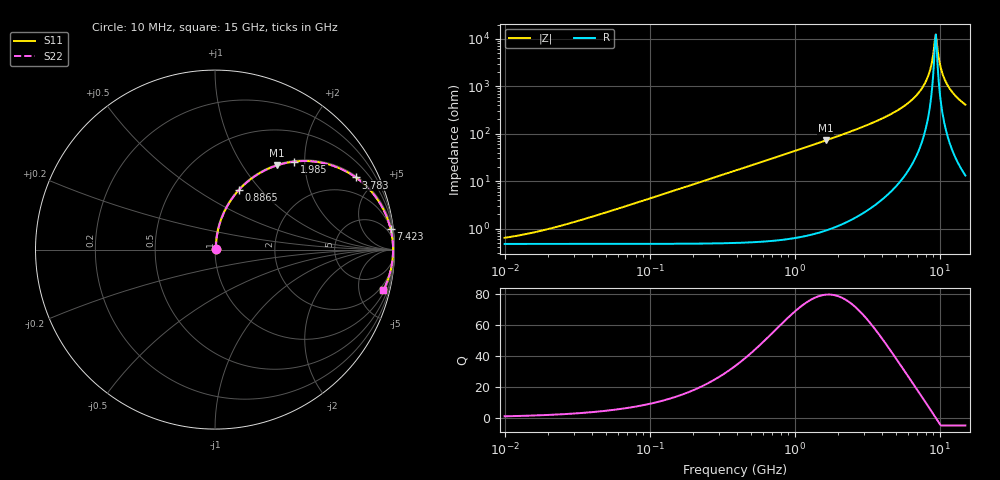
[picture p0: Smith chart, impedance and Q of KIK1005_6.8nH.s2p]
!version-3
!date-01.2023
!Series
# Hz S RI R 50
!Freq ReS11 ImS11 ReS21 ImS21 ReS12 ImS12 ReS22 ImS22
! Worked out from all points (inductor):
!   500 points, 10 MHz to 15 GHz, reference 50 ohm
!   read as one part in series: L = 6.8 nH near 33.75 MHz
!   highest Q = 79.5 at 1.641 GHz (marker M1), where L = 7.01 nH
!   self-resonance near 9.248 GHz
!   S11 on the Smith chart (normalised r, x): 10 MHz: 1.01, +0.01; 886.5 MHz: 1.01, +0.76; 1.985 GHz: 1.02, +1.78; 3.783 GHz: 1.07, +3.86; 7.423 GHz: 2, +17; 15 GHz: 1.26, -8.18
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1e7  0.00474 0.00423  0.9953 -0.00423  0.9953 -0.00423  0.00474 0.00423
3.424937e7  0.00493 0.0145  0.9951 -0.0145  0.9951 -0.0145  0.00493 0.0145
1.155953e8  0.00714 0.0488  0.9929 -0.0488  0.9929 -0.0488  0.00714 0.0488
3.901468e8  0.0317 0.1609  0.9683 -0.1609  0.9683 -0.1609  0.0317 0.1609
8.864682e8  0.1313 0.33  0.8687 -0.33  0.8687 -0.33  0.1313 0.33
1.316788e9  0.2506 0.4269  0.7494 -0.4269  0.7494 -0.4269  0.2506 0.4269
1.64055e9  0.3452 0.4692  0.6548 -0.4692  0.6548 -0.4692  0.3452 0.4692
1.984876e9  0.4416 0.4903  0.5584 -0.4903  0.5584 -0.4903  0.4416 0.4903
3.782592e9  0.7842 0.4022  0.2158 -0.4022  0.2158 -0.4022  0.7842 0.4022
4.444302e9  0.8517 0.3444  0.1483 -0.3444  0.1483 -0.3444  0.8517 0.3444
6.04598e9  0.9443 0.2114  0.0557 -0.2114  0.0557 -0.2114  0.9443 0.2114
7.422932e9  0.9786 0.1138  0.0214 -0.1138  0.0214 -0.1138  0.9786 0.1138
7.987301e9  0.9857 0.0781  0.0143 -0.0781  0.0143 -0.0781  0.9857 0.0781
8.469537e9  0.9895 0.0494  0.0105 -0.0494  0.0105 -0.0494  0.9895 0.0494
8.850227e9  0.9912 0.0278  0.00878 -0.0278  0.00878 -0.0278  0.9912 0.0278
9.11348e9  0.9918 0.0134  0.00817 -0.0134  0.00817 -0.0134  0.9918 0.0134
9.384563e9  0.992 -0.000988  0.00797 0.000988  0.00797 0.000988  0.992 -0.000988
9.523114e9  0.992 -0.0082  0.00803 0.0082  0.00803 0.0082  0.992 -0.0082
1.024716e10  0.9901 -0.0442  0.00989 0.0442  0.00989 0.0442  0.9901 -0.0442
1.102626e10  0.9856 -0.0801  0.0144 0.0801  0.0144 0.0801  0.9856 -0.0801
1.258092e10  0.9708 -0.1441  0.0292 0.1441  0.0292 0.1441  0.9708 -0.1441
1.5e10  0.9372 -0.2271  0.0628 0.2271  0.0628 0.2271  0.9372 -0.2271
